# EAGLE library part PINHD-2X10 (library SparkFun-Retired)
PIN HEADER
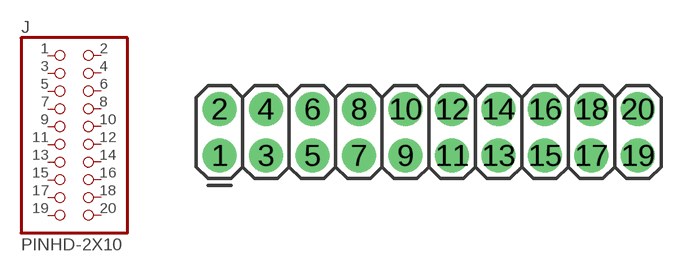
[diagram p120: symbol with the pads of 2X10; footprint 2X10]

Designator prefix J

## PINHD-2X10  [2X10]
1  1  pas
2  2  pas
3  3  pas
4  4  pas
5  5  pas
6  6  pas
7  7  pas
8  8  pas
9  9  pas
10  10  pas
11  11  pas
12  12  pas
13  13  pas
14  14  pas
15  15  pas
16  16  pas
17  17  pas
18  18  pas
19  19  pas
20  20  pas

## Footprint 2X10 (pad centres in mm)
PIN HEADER
drill 1.016 pad 1.88: 1 0,0; 2 0,2.54; 3 2.54,0; 4 2.54,2.54; 5 5.08,0; 6 5.08,2.54; 7 7.62,0; 8 7.62,2.54; 9 10.16,0; 10 10.16,2.54; 11 12.7,0; 12 12.7,2.54; 13 15.24,0; 14 15.24,2.54; 15 17.78,0; 16 17.78,2.54; 17 20.32,0; 18 20.32,2.54; 19 22.86,0; 20 22.86,2.54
